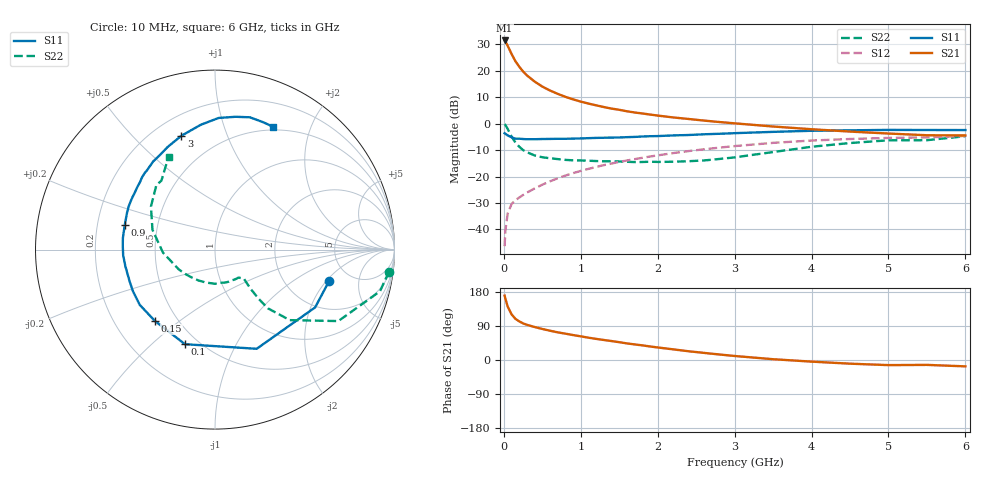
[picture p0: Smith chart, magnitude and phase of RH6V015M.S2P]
! SIEMENS Small Signal Semiconductors
! BFR106
! Si NPN RF Bipolar Junction Transistor in SOT23
! VCE = 6 V  IC = 15 mA
! Common Emitter S-Parameters:  August  1996
# GHz  S  MA  R  50
!  f  S11  S21  S12  S22
! GHz  MAG  ANG  MAG  ANG  MAG  ANG  MAG  ANG
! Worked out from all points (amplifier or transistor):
!   36 points, 10 MHz to 6 GHz, reference 50 ohm
!   highest |S21| = 31.5 dB at 10 MHz (marker M1)
!   |S21| within 3 dB of that: start of sweep to 66.23 MHz
!   unconditionally stable (mu >= 1): 413.7 MHz to 2.043 GHz
!   at 250 MHz: K = 0.82, MSG = 23.4 dB, |S12| = -27.0 dB
!   at 1.4 GHz: K = 1.08, MAG = 8.7 dB, |S12| = -15.1 dB
!   at 6 GHz: K = 1.00, MSG = 0.1 dB, |S12| = -4.7 dB
!   S11 on the Smith chart (normalised r, x): 10 MHz: 3.45, -2.15; 100 MHz: 0.42, -0.64; 150 MHz: 0.38, -0.41; 900 MHz: 0.32, +0.12; 3 GHz: 0.31, +0.70; 6 GHz: 0.46, +1.47
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0.01  0.6592 -15.5  37.63 170.0  0.0048 82.7  0.9772 -7.2
0.02  0.6442 -30.0  36.26 162.1  0.0095 80.2  0.948 -14.2
0.05  0.5995 -67.2  29.92 140.9  0.0199 64.0  0.7941 -30.1
0.1  0.553 -107.6  20.91 120.6  0.0301 53.8  0.573 -43.3
0.15  0.5198 -130.1  15.28 108.7  0.0356 51.0  0.44 -48.0
0.2  0.5201 -143.7  11.99 101.9  0.04 52.7  0.367 -48.4
0.25  0.5125 -153.0  9.733 96.6  0.0447 53.9  0.3164 -48.0
0.3  0.5077 -159.4  8.211 92.9  0.0496 56.6  0.2886 -47.6
0.4  0.508 -169.6  6.272 87.0  0.0594 59.5  0.2504 -46.2
0.5  0.5127 -176.6  5.042 81.9  0.07 62.0  0.2314 -45.3
0.6  0.5144 177.4  4.242 77.3  0.081 63.5  0.2218 -46.1
0.7  0.5173 172.7  3.67 73.0  0.0926 64.5  0.2137 -47.7
0.9  0.5213 164.7  2.886 65.8  0.116 65.1  0.2026 -51.0
1.1  0.5321 156.9  2.403 58.9  0.1396 64.6  0.199 -57.1
1.3  0.5415 150.1  2.064 52.8  0.1643 63.6  0.1943 -63.4
1.6  0.5556 141.2  1.716 43.8  0.2009 61.2  0.1901 -75.7
2.2  0.5997 125.1  1.314 28.1  0.2772 54.8  0.1903 -105.0
3  0.6613 106.4  1.016 10.6  0.3763 43.6  0.2303 -151.5
3.5  0.7 96.5  0.884 2.1  0.4336 35.8  0.2904 -176.7
4.5  0.7488 81.2  0.709 -9.7  0.5128 19.3  0.4301 146.1
5.5  0.7587 69.2  0.604 -12.9  0.5498 8.1  0.4868 127.8
6  0.7572 64.9  0.599 -16.8  0.585 0.3  0.5792 116.5
